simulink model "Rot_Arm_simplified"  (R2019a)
settings: Solver=ode4  StartTime=0.0  StopTime=2  FixedStep=0.01  RelTol=1e-3  EnableMultiTasking=on
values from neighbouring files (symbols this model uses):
  g = 9.81    [Parameters_Rot_Arm.m]
  J_t = 5E-04    (= 0.0005)    [Parameters_Rot_Arm.m]
  K_t = 0.0538    [Parameters_Rot_Arm.m]
  K_vis = 3E-4    (= 0.0003)    [Parameters_Rot_Arm.m]
  l = 0.1    [Parameters_Rot_Arm.m]
  M = 0.01    [Parameters_Rot_Arm.m]
  Mb = 0.025    [Parameters_Rot_Arm.m]
libraries: simulink_extras x2

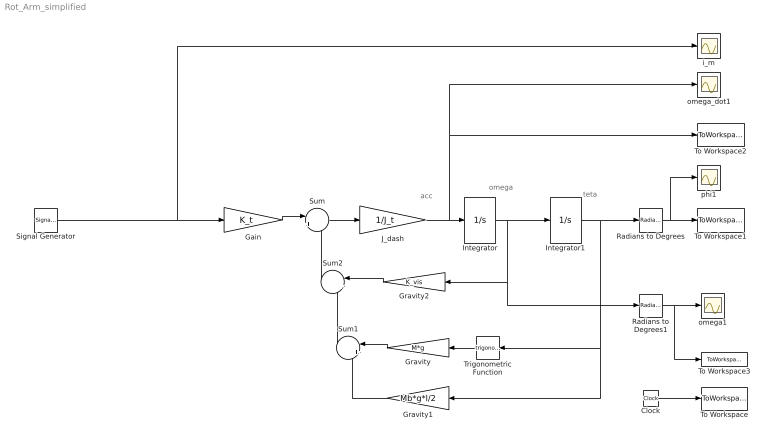
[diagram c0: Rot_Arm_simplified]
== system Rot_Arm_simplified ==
  note: acc
  note: omega
  note: teta
  Clock : Clock
  Gain : Gain  Gain=K_t
  Gravity : Gain  Gain=M*g
  Gravity1 : Gain  Gain=Mb*g*l/2
  Gravity2 : Gain  Gain=K_vis
  Integrator : Integrator
  Integrator1 : Integrator
  J_dash : Gain  Gain=1/J_t
  Radians to Degrees : simulink_extras/Transformations/Radians to Degrees
  Radians to Degrees1 : simulink_extras/Transformations/Radians to Degrees
  Signal Generator : SignalGenerator  WaveForm=square
  Sum : Sum  Inputs=|+-
  Sum1 : Sum  Inputs=|++
  Sum2 : Sum  Inputs=|++
  To Workspace : ToWorkspace  VariableName=t  SampleTime=-1
  To Workspace1 : ToWorkspace  VariableName=phi  SampleTime=-1
  To Workspace2 : ToWorkspace  VariableName=omega_dot  SampleTime=-1
  To Workspace3 : ToWorkspace  VariableName=omega  SampleTime=-1
  Trigonometric Function : Trigonometry
  i_m : Scope
  omega1 : Scope
  omega_dot1 : Scope
  phi1 : Scope
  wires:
  Integrator/1 -> Integrator1/1, Radians to Degrees1/1, Gravity2/1
  J_dash/1 -> omega_dot1/1, To Workspace2/1, Integrator/1
  Trigonometric Function/1 -> Gravity/1
  Radians to Degrees/1 -> phi1/1, To Workspace1/1
  Clock/1 -> To Workspace/1
  Radians to Degrees1/1 -> To Workspace3/1, omega1/1
  Signal Generator/1 -> i_m/1, Gain/1
  Gravity1/1 -> Sum1/2
  Gravity/1 -> Sum1/1
  Gravity2/1 -> Sum2/1
  Sum1/1 -> Sum2/2
  Sum2/1 -> Sum/2
  Gain/1 -> Sum/1
  Sum/1 -> J_dash/1
  Integrator1/1 -> Gravity1/1, Trigonometric Function/1, Radians to Degrees/1
